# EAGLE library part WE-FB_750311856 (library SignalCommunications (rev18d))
WE-FB Flyback Transformer suitable for LT3573/ LT3574/ LT3575/ LT3748 Characteristics easy design in solution less external components needed small board space low cost no optocoupler needed! long term reliability voltage control no aging same external parts for different output voltages easy design of custom power supply due to standard circuit and change of transformers and two components for feedback loop Isolation voltage up to 2.5 kV Applications Isolated power design Sensor interfaces Isolated telecom converters Power over Ethernet Details see: http://katalog.we-online.de/en/pbs/WE-FB_Linear? Updated 2014-07-07 2014 (C) Wurth Elektronik
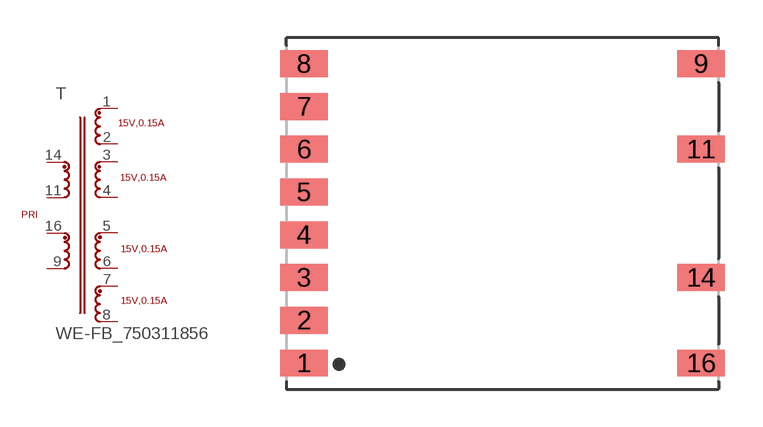
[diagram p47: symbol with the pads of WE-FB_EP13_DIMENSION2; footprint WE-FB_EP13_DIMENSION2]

Designator prefix T

## WE-FB_750311856  [WE-FB_EP13_DIMENSION2]
1  2  pas
2  3  pas
3  4  pas
4  5  pas
5  6  pas
6  7  pas
7  8  pas
8  9  pas
9  10  pas
11  12  pas
14  1  pas
16  11  pas

## Footprint WE-FB_EP13_DIMENSION2 (pad centres in mm)
smd 1.88 x 1.07: 1 -7.885,-5.95; 2 -7.885,-4.25; 3 -7.885,-2.55; 4 -7.885,-0.85; 5 -7.885,0.85; 6 -7.885,2.55; 7 -7.885,4.25; 8 -7.885,5.95; 9 7.885,5.95; 11 7.885,2.55; 14 7.885,-2.55; 16 7.885,-5.95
